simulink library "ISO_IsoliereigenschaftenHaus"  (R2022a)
settings: Solver=VariableStepAuto  StartTime=0.0  StopTime=10.0  RelTol=1e-3
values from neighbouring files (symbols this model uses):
  PAR_ISO_BodenUWert = 0.073    [parameter_ISO.m]
  PAR_ISO_DachUWert = 0.188    [parameter_ISO.m]
  PAR_ISO_FensterUWert = 0.5    [parameter_ISO.m]
  PAR_ISO_WaendeUWert = 0.187    [parameter_ISO.m]
  PAR_ISO_WarmekapazitaetBoden = 63    [parameter_ISO.m]
  PAR_ISO_WarmekapazitaetDach = 448    [parameter_ISO.m]
  PAR_ISO_WarmekapazitaetFenster = 21.6    [parameter_ISO.m]
  PAR_ISO_WarmekapazitaetWand = 353    [parameter_ISO.m]

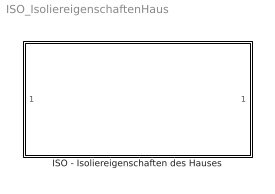
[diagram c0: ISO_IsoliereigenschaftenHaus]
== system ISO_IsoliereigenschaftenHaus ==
  ISO - Isoliereigenschaften des Hauses : Subsystem

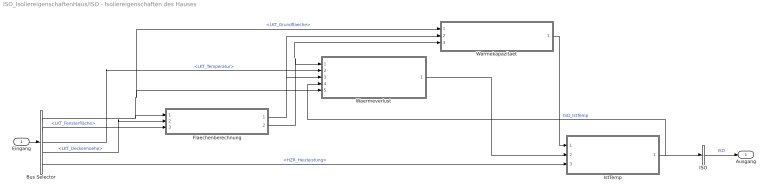
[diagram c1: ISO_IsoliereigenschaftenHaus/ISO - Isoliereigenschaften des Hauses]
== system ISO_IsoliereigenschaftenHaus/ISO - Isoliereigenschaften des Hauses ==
  Eingang : Inport
  Bus Selector : BusSelector  OutputSignals=LKT_Grundflaeche,LKT_Fensterfläche,LKT_Temperatur,LKT_Deckenhoehe,HZR_Heizleistung
  Flaechenberechnung : Subsystem
  ISO : BusCreator  Inputs=1
  IstTemp : Subsystem
  Waermeverlust : Subsystem
  Warmekapazitaet : Subsystem
  Ausgang : Outport
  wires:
  Waermeverlust/1(ISO_Waermeverlust) -> IstTemp/2(ISO_Waermeverlust)
  Flaechenberechnung/2(ISO_FlaecheFenster) -> Warmekapazitaet/3(ISO_FlaecheFenster), Waermeverlust/1(ISO_Flaeche_Fenster)
  Flaechenberechnung/1(ISO_FlaecheWand) -> Warmekapazitaet/2(ISO_FlaecheWand), Waermeverlust/3(ISO_FlaecheWand)
  Eingang/1 -> Bus Selector/1
  Warmekapazitaet/1(ISO_Waermekapazitaet) -> IstTemp/1(ISO_Warmekapazitaet)
  ISO/1 -> Ausgang/1  "ISO"
  Bus Selector/1 -> Flaechenberechnung/1(<LKT_Grundflaeche>), Warmekapazitaet/1(LKT_Grundflaeche), Waermeverlust/5(LKT_Grundflaeche)  "<LKT_Grundflaeche>"
  Bus Selector/3 -> Waermeverlust/2(LKT_Temperatur)  "<LKT_Temperatur>"
  Bus Selector/4 -> Flaechenberechnung/2(<LKT_Deckenhoehe>)  "<LKT_Deckenhoehe>"
  IstTemp/1(ISO_IstTemp) -> Waermeverlust/4(ISO_IstTemp), ISO/1  "ISO_IstTemp"
  Bus Selector/2 -> Flaechenberechnung/3(<LKT_Fensterfläche>)  "<LKT_Fensterfläche>"
  Bus Selector/5 -> IstTemp/3(HZR_Heizleistung)  "<HZR_Heizleistung>"

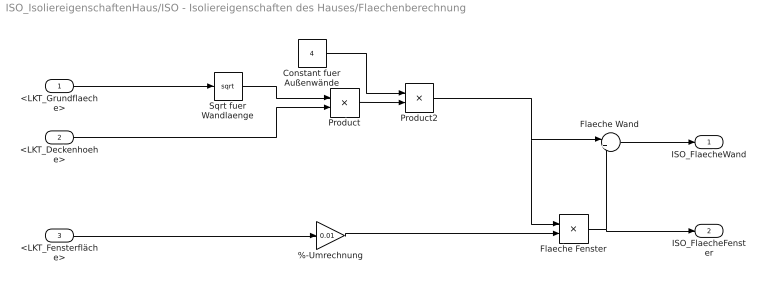
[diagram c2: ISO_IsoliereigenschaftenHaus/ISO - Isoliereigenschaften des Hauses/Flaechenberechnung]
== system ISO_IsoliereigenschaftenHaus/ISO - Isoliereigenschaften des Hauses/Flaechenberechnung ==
  <LKT_Grundflaeche> : Inport
  <LKT_Deckenhoehe> : Inport  Port=2
  <LKT_Fensterfläche> : Inport  Port=3
  %-Umrechnung : Gain  Gain=0.01
  Constant fuer Außenwände : Constant  Value=4
  Flaeche Fenster : Product
  "Flaeche Wand " : Sum  Inputs=|+-
  Product : Product
  Product2 : Product
  Sqrt fuer Wandlaenge : Sqrt
  ISO_FlaecheWand : Outport  VectorParamsAs1DForOutWhenUnconnected=off
  ISO_FlaecheFenster : Outport  Port=2  VectorParamsAs1DForOutWhenUnconnected=off
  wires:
  <LKT_Grundflaeche>/1 -> Sqrt fuer Wandlaenge/1
  Sqrt fuer Wandlaenge/1 -> Product/1
  <LKT_Deckenhoehe>/1 -> Product/2
  Product2/1 -> Flaeche Fenster/1, "Flaeche Wand "/1
  Product/1 -> Product2/2
  Constant fuer Außenwände/1 -> Product2/1
  Flaeche Fenster/1 -> ISO_FlaecheFenster/1, "Flaeche Wand "/2
  "Flaeche Wand "/1 -> ISO_FlaecheWand/1
  <LKT_Fensterfläche>/1 -> %-Umrechnung/1
  %-Umrechnung/1 -> Flaeche Fenster/2

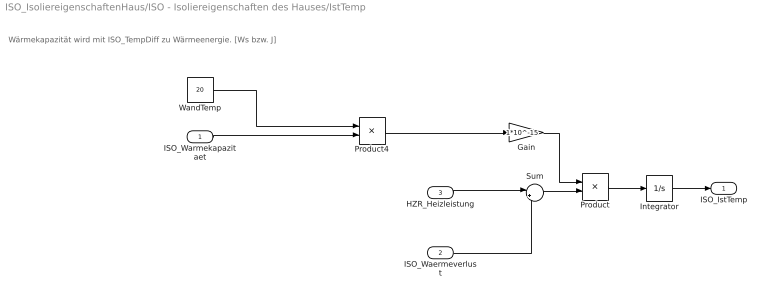
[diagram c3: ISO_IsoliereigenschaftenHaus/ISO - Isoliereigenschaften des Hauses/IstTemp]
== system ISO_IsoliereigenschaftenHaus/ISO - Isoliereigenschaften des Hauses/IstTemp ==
  note: Wärmekapazität wird mit ISO_TempDiff zu Wärmeenergie. [Ws bzw. J]
  ISO_Warmekapazitaet : Inport
  ISO_Waermeverlust : Inport  Port=2
  HZR_Heizleistung : Inport  Port=3
  Gain : Gain  Gain=1*10^-15
  Integrator : Integrator  InitialCondition=20
  Product : Product
  Product4 : Product
  Sum : Sum  Inputs=|++
  WandTemp : Constant  Value=20
  ISO_IstTemp : Outport
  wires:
  Product/1 -> Integrator/1
  Integrator/1 -> ISO_IstTemp/1
  HZR_Heizleistung/1 -> Sum/1
  ISO_Waermeverlust/1 -> Sum/2
  Sum/1 -> Product/2
  Gain/1 -> Product/1
  WandTemp/1 -> Product4/1
  ISO_Warmekapazitaet/1 -> Product4/2
  Product4/1 -> Gain/1

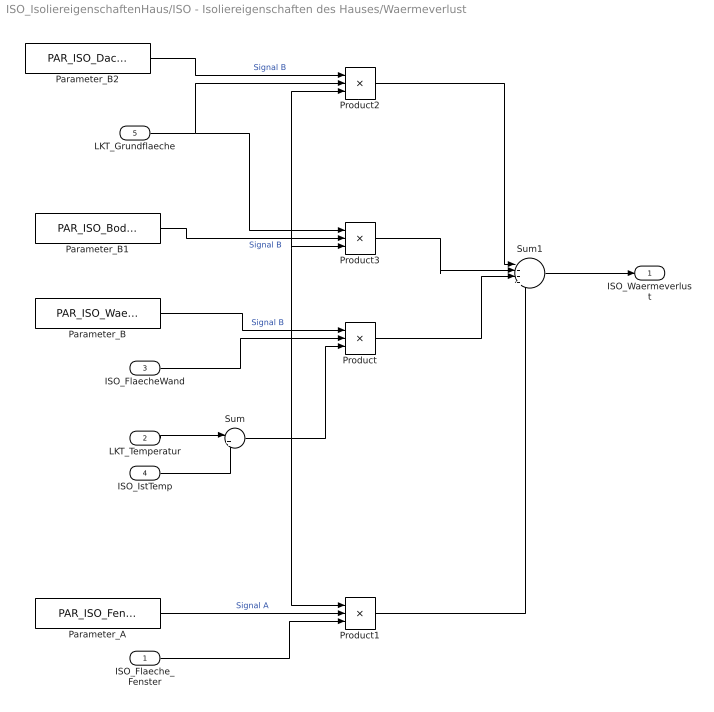
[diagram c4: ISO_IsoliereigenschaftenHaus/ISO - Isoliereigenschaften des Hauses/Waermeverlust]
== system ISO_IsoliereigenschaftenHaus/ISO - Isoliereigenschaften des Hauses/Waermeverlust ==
  ISO_Flaeche_Fenster : Inport
  LKT_Temperatur : Inport  Port=2
  ISO_FlaecheWand : Inport  Port=3
  ISO_IstTemp : Inport  Port=4
  LKT_Grundflaeche : Inport  Port=5
  Parameter_A : Constant  Value=PAR_ISO_FensterUWert
  Parameter_B : Constant  Value=PAR_ISO_WaendeUWert
  Parameter_B1 : Constant  Value=PAR_ISO_BodenUWert
  Parameter_B2 : Constant  Value=PAR_ISO_DachUWert
  Product{,1..3} (4 alike) : Product  Inputs=3
  Sum : Sum  Inputs=|+-
  Sum1 : Sum  Inputs=|++++
  ISO_Waermeverlust : Outport
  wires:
  LKT_Temperatur/1 -> Sum/1
  ISO_IstTemp/1 -> Sum/2
  Parameter_B/1 -> Product/1  "Signal B"
  ISO_FlaecheWand/1 -> Product/2
  Sum/1 -> Product/3, Product1/1, Product3/3, Product2/3
  Parameter_A/1 -> Product1/2  "Signal A"
  ISO_Flaeche_Fenster/1 -> Product1/3
  Product/1 -> Sum1/3
  Product1/1 -> Sum1/4
  Sum1/1 -> ISO_Waermeverlust/1
  Parameter_B2/1 -> Product2/1  "Signal B"
  LKT_Grundflaeche/1 -> Product2/2, Product3/1
  Parameter_B1/1 -> Product3/2  "Signal B"
  Product3/1 -> Sum1/2
  Product2/1 -> Sum1/1

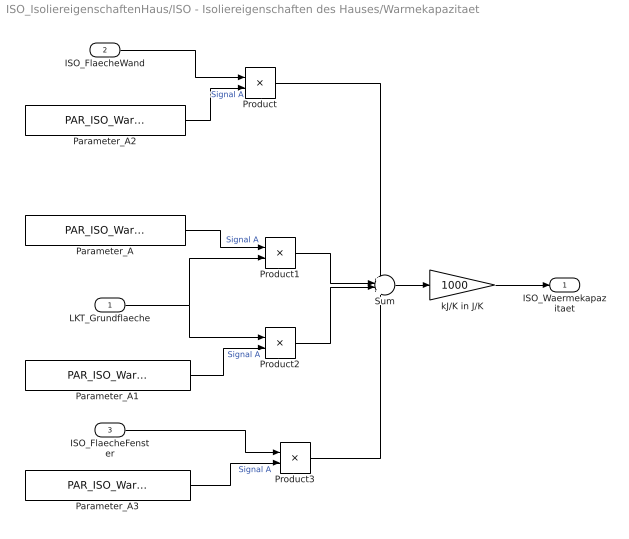
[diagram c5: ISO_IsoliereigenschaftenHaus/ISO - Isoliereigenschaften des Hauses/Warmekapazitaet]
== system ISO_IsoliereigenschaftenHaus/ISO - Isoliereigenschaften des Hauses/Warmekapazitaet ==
  LKT_Grundflaeche : Inport
  ISO_FlaecheWand : Inport  Port=2
  ISO_FlaecheFenster : Inport  Port=3
  Parameter_A : Constant  Value=PAR_ISO_WarmekapazitaetDach
  Parameter_A1 : Constant  Value=PAR_ISO_WarmekapazitaetBoden
  Parameter_A2 : Constant  Value=PAR_ISO_WarmekapazitaetWand
  Parameter_A3 : Constant  Value=PAR_ISO_WarmekapazitaetFenster
  Product{,1..3} (4 alike) : Product
  Sum : Sum  Inputs=++++
  kJ/K in J/K : Gain  Gain=1000
  ISO_Waermekapazitaet : Outport
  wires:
  LKT_Grundflaeche/1 -> Product1/2, Product2/1
  Parameter_A/1 -> Product1/1  "Signal A"
  ISO_FlaecheFenster/1 -> Product3/1
  Parameter_A3/1 -> Product3/2  "Signal A"
  Parameter_A1/1 -> Product2/2  "Signal A"
  Parameter_A2/1 -> Product/2  "Signal A"
  ISO_FlaecheWand/1 -> Product/1
  Product/1 -> Sum/1
  Product1/1 -> Sum/2
  Product2/1 -> Sum/3
  Product3/1 -> Sum/4
  kJ/K in J/K/1 -> ISO_Waermekapazitaet/1
  Sum/1 -> kJ/K in J/K/1
